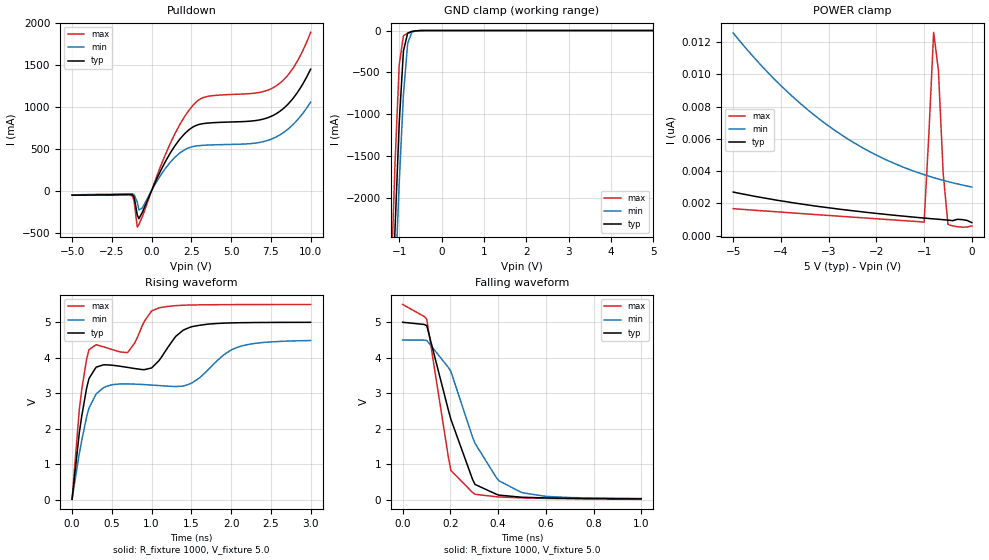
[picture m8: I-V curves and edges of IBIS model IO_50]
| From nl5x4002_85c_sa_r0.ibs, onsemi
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[Model]   IO_50
Model_type I/O_open_drain
Enable Active-High
Polarity Non-Inverting
Vinh=3.5
Vinl=1.5
Vref=5.0
Vmeas=2.5
Rref=1000
Cref=50p
C_comp   6.0p   NA   NA
[Model Spec]
Vinh   3.5   3.15   3.85
Vinl   1.5   1.35   1.65
Vmeas   2.5   2.25   2.75
[Temperature Range] 25   85   -40
[Voltage Range]   5.0   4.5   5.5
[POWER Clamp Reference]  5.0   4.5   5.5
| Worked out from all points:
|   slope of the pulldown table from 0 to 0.75 V, typ, clamps not added: 2.47 ohm
|   GND clamp passes 1 mA (typ) near -0.51 V on its own axis
|   falling waveform, R_fixture 1000, V_fixture 5.0: 20-80 % time 134ps typ, 162ps min, 77.2ps max; typ from 5 V to 0.03 V
|   rising waveform, R_fixture 1000, V_fixture 5.0: 20-80 % time 1.07ns typ, 1.62ns min, 743ps max; typ from 0.011 V to 5 V
[Pulldown]
-5V       -55.3mA    -51.31mA   -55.54mA
-1.2V     -50.45mA   -38.38mA   -67.45mA
-1.1V     -76.97mA   -49.95mA   -125.5mA
-900mV    -291mA     -138.4mA   -436mA
-800mV    -335.1mA   -229.9mA   -404.8mA
-600mV    -264.8mA   -211mA     -318.7mA
1.2V      455.3mA    342.5mA    572.3mA
2.6V      757.8mA    524.8mA    1.016A
3.5V      803.8mA    542.1mA    1.121A
7.7V      901.6mA    627mA      1.232A
8.9V      1.1A       788.5mA    1.461A
10V       1.447A     1.054A     1.886A
[GND Clamp]
-5V       -61.05A    -56.68A    -66.63A
-1.2V     -3.822A    -4.412A    -3.136A
-1.1V     -2.385A    -3.071A    -1.6A
-1V       -1.105A    -1.818A    -410.1mA
-900mV    -244.1mA   -763.4mA   -62.39mA
-800mV    -31.41mA   -154.3mA   -31.83mA
-700mV    -10.05mA   -17.99mA   -15.56mA
-600mV    -3.32mA    -2.981mA   -4.628mA
5V        807.9pA    3.009nA    603.3pA
[POWER Clamp]
-5V       2.7nA      12.56nA    1.671nA
-4V       2.156nA    9.294nA    1.46nA
-3.1V     1.765nA    7.011nA    1.271nA
-2.1V     1.409nA    5.144nA    1.069nA
-1V       1.09nA     3.779nA    834.5pA
-900mV    1.064nA    3.686nA    6.293nA
-800mV    1.038nA    3.597nA    12.6nA
-700mV    1.013nA    3.51nA     10.25nA
-600mV    988.5pA    3.427nA    3.857nA
-500mV    963.9pA    3.35nA     693.6pA
-200mV    992.9pA    3.14nA     526.2pA
0V        807pA      3.009nA    603.3pA
[Falling Waveform]
R_fixture=1000
V_fixture=5.0
V_fixture_min=4.5
V_fixture_max=5.5
0s        5V         4.5V       5.5V
101ps     4.905V     4.488V     5.083V
191.9ps   2.52V      3.725V     1.19V
202ps     2.27V      3.616V     830.7mV
292.9ps   578.6mV    1.771V     209mV
303ps     437.6mV    1.595V     158.3mV
404ps     135.1mV    536.9mV    83.43mV
494.9ps   78.44mV    221mV      59.55mV
606.1ps   55.59mV    98.57mV    43.1mV
1ns       29.95mV    40.61mV    17.07mV
[Rising Waveform]
R_fixture=1000
V_fixture=5.0
V_fixture_min=4.5
V_fixture_max=5.5
0s        11.17mV    12.77mV    10.13mV
90.91ps   1.888V     1.304V     2.544V
212.1ps   3.411V     2.58V      4.225V
393.9ps   3.799V     3.154V     4.308V
697ps     3.728V     3.263V     4.144V
1ns       3.711V     3.23V      5.317V
1.121ns   4.006V     3.212V     5.418V
1.515ns   4.879V     3.301V     5.487V
2.091ns   4.986V     4.304V     5.497V
3ns       4.998V     4.485V     5.5V
[Ramp]
R_load=1000
dV/dt_r   2.993E+0/1.333E-10   2.692E+0/1.681E-10   3.187E+0/6.988E-10
dV/dt_f   2.982E+0/1.337E-10   2.676E+0/1.621E-10   3.290E+0/7.683E-11
|[End   IO_50
